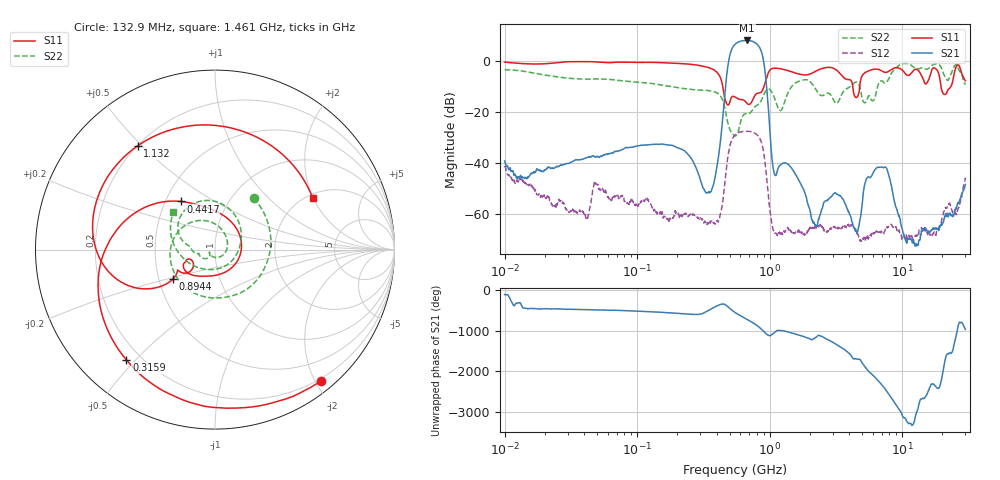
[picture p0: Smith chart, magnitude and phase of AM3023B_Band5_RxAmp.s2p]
# Hz S DB R 50.0
!freq dBS11 angS11 dBS21 angS21 dBS12 angS12 dBS22 angS22
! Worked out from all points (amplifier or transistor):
!   1601 points, 10 MHz to 30 GHz, reference 50 ohm
!   highest |S21| = 8.0 dB at 675.8 MHz (marker M1)
!   |S21| within 3 dB of that: 522.5 MHz to 844.7 MHz (322.2 MHz wide, 47.1 % of centre)
!   unconditionally stable (mu >= 1): start of sweep to end of sweep
!   at 37.85 MHz: K = 1468.86, MAG = -24.8 dB, |S12| = -58.3 dB
!   at 547.7 MHz: K = 6.44, MAG = 6.7 dB, |S12| = -29.0 dB
!   at 30 GHz: K = 18364.52, MAG = -47.0 dB, |S12| = -45.6 dB
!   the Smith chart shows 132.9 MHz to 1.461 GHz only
!   S11 on the Smith chart (normalised r, x): 132.9 MHz: 0.16, -2.08; 315.9 MHz: 0.15, -0.47; 441.7 MHz: 0.60, +0.36; 894.4 MHz: 0.59, -0.21; 1.132 GHz: 0.20, +0.49; 1.461 GHz: 2.14, +1.98
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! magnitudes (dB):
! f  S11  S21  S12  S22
! 10 MHz  -0.4  -39.1  -41.1  -3.4
! 38.04 MHz  -0.2  -38.6  -58.6  -7.1
! 48.85 MHz  -0.4  -37.6  -48.3  -7.0
! 132.9 MHz  -0.5  -32.6  -57.7  -8.9
! 144.7 MHz  -0.6  -32.6  -59.4  -9.2
! 315.9 MHz  -2.1  -49.8  -62.5  -11.4
! 374.5 MHz  -3.3  -48.8  -62.8  -11.9
! 441.7 MHz  -9.6  -22.8  -55.4  -15.4
! 547.7 MHz  -14.1  6.5  -29.0  -29.4
! 675.8 MHz  -16.6  8.0  -27.5  -20.7
! 894.4 MHz  -10.8  0.7  -34.8  -13.8
! 1.055 GHz  -2.9  -40.8  -65.5  -12.9
! 1.132 GHz  -2.8  -43.9  -67.7  -17.1
! 1.461 GHz  -4.2  -41.9  -67.1  -10.1
! 2.084 GHz  -4.8  -62.2  -65.5  -8.9
! 3.172 GHz  -3.4  -51.9  -65.6  -16.6
! 4.548 GHz  -14.2  -67.3  -67.4  -8.3
! 5.419 GHz  -4.2  -45.9  -68.7  -15.4
! 7.926 GHz  -4.0  -44.7  -64.7  -7.0
! 10.44 GHz  -4.6  -69.3  -68.8  -0.9
! 12.75 GHz  -3.2  -71.5  -68.3  -3.0
! 30 GHz  -7.7  -48.4  -45.6  -9.3
